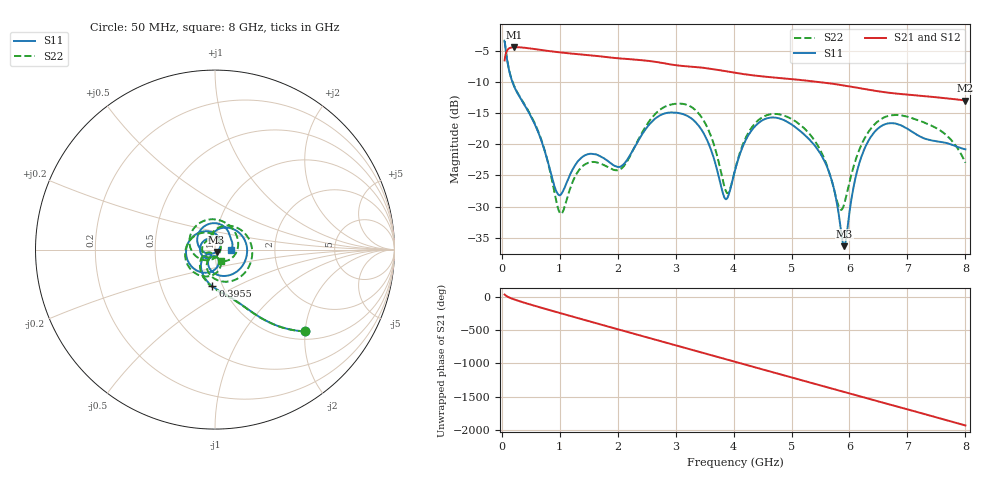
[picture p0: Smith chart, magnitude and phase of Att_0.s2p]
#  HZ  S  DB  R  50.00
! Rohde & Schwarz Vector Network Analyzer
! Rohde-Schwarz,ZNB40-4Port,1311601084101679,3.45
! Created: UTC 4/25/2025, 9:26:08 AM
! freq[Hz]  db:S11  ang:S11  db:S21  ang:S21  db:S12  ang:S12  db:S22  ang:S22
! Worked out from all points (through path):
!   1750 points, 50 MHz to 8 GHz, reference 50 ohm
!   highest |S21| = -4.43 dB at 218.2 MHz (marker M1); lowest = -13.0 dB at 8 GHz (marker M2)
!   group delay of S21, straight-line fit = 668 ps
!   lowest |S11| = -36.4 dB at 5.909 GHz (marker M3), VSWR 1.03, Z = 50.9 - j1.27 ohm
!   |S11| at or under -10 dB: 183.8 MHz to end of sweep
!   |S22| runs from -31.2 to -3.4 dB; largest |S21 - S12| = 0.00077
!   S11 on the Smith chart (normalised r, x): 50 MHz: 1.19, -1.99; 395.5 MHz: 0.89, -0.38; 8 GHz: 1.20, -0.00
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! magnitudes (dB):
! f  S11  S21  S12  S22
! 50 MHz  -3.4  -6.6  -6.6  -3.4
! 218.2 MHz  -10.8  -4.4  -4.4  -10.7
! 395.5 MHz  -13.7  -4.5  -4.5  -13.7
! 700 MHz  -19.9  -4.9  -4.9  -19.8
! 1.009 GHz  -28.2  -5.3  -5.3  -31.1
! 1.377 GHz  -22.2  -5.6  -5.6  -23.7
! 2.059 GHz  -23.5  -6.3  -6.3  -24.0
! 2.7 GHz  -15.6  -6.9  -6.9  -14.7
! 3.395 GHz  -17.0  -7.7  -7.7  -15.0
! 3.627 GHz  -21.3  -7.9  -7.9  -19.1
! 3.859 GHz  -28.8  -8.3  -8.3  -27.3
! 4.027 GHz  -24.1  -8.6  -8.6  -24.0
! 4.25 GHz  -18.7  -8.9  -8.9  -18.3
! 4.545 GHz  -16.0  -9.2  -9.2  -15.5
! 5.35 GHz  -19.7  -9.9  -9.9  -18.8
! 5.668 GHz  -25.0  -10.3  -10.3  -25.0
! 5.823 GHz  -31.7  -10.5  -10.5  -30.2
! 5.909 GHz  -36.4  -10.6  -10.6  -29.6
! 6.223 GHz  -21.6  -11.1  -11.1  -19.8
! 6.677 GHz  -16.6  -11.7  -11.7  -15.4
! 7.523 GHz  -19.6  -12.5  -12.5  -17.5
! 8 GHz  -20.8  -13.0  -13.0  -23.0
